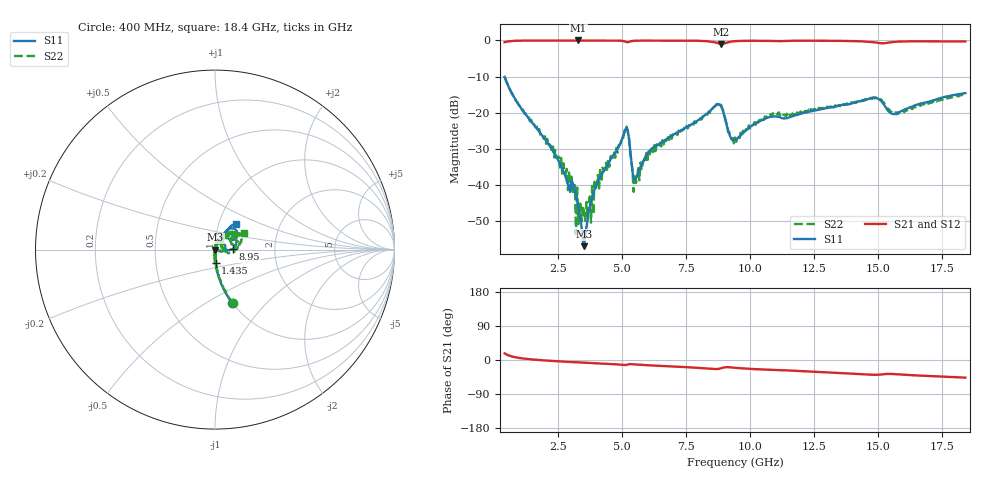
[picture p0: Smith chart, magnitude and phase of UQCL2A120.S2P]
! AVX Corporation
! Date:  10/27/06
! Part No:  UQCL2A120
! Description:  Ultra Low ESR Microwave capacitors
! Mounting Orientation:  Horizontal
# GHZ S DB R 50
! Freq  |S11|  S11 Ph  |S21|  S21 Ph  |S12|  S12 Ph  |S22|  S22 Ph
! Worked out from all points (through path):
!   401 points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, 400 MHz to 18.4 GHz, reference 50 ohm
!   highest |S21| = -0.02 dB at 3.28 GHz (marker M1); lowest = -1.0 dB at 8.86 GHz (marker M2)
!   group delay of S21, straight-line fit = 7.75 ps
!   lowest |S11| = -57.0 dB at 3.505 GHz (marker M3), VSWR 1.00, Z = 50.1 - j0.0112 ohm
!   |S11| at or under -10 dB: start of sweep to end of sweep
!   |S22| runs from -53.7 to -10.0 dB; largest |S21 - S12| = 0.0033
!   S11 on the Smith chart (normalised r, x): 400 MHz: 1.00, -0.66; 1.435 GHz: 1.00, -0.15; 8.95 GHz: 1.22, +0.01; 18.4 GHz: 1.21, +0.36
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0.4  -10.11 -72.1  -0.49 17.5  -0.48 17.4  -10.03 -71.0
1.435  -22.43 -87.4  -0.04 1.7  -0.03 1.7  -21.98 -87.6
2.695  -36.15 -91.3  -0.02 -4.2  -0.01 -4.2  -34.02 -94.8
2.875  -39.84 -98.1  -0.02 -4.9  -0.01 -4.9  -41.47 -87.0
3.1  -40.20 -86.7  -0.03 -5.7  -0.02 -5.7  -42.53 -126.5
3.28  -45.98 -81.4  -0.02 -6.3  -0.02 -6.3  -50.87 -14.1
3.415  -52.16 -62.8  -0.03 -6.8  -0.02 -6.8  -50.16 -179.6
3.505  -56.98 -4.5  -0.02 -7.1  -0.02 -7.1  -47.63 91.4
3.955  -40.70 67.0  -0.03 -8.5  -0.03 -8.6  -40.91 111.9
5.125  -24.55 35.0  -0.36 -13.3  -0.35 -13.4  -25.18 42.3
5.215  -25.08 1.3  -0.50 -11.7  -0.50 -11.8  -25.74 8.8
5.485  -38.65 23.5  -0.10 -11.9  -0.10 -11.9  -37.05 23.8
6.43  -28.71 66.9  -0.05 -15.4  -0.05 -15.4  -28.99 66.8
8.86  -18.32 13.6  -0.99 -21.7  -1.00 -21.8  -17.85 4.0
8.95  -20.01 2.3  -0.92 -19.9  -0.92 -20.0  -19.59 -9.2
9.22  -26.71 10.6  -0.36 -19.5  -0.37 -19.6  -27.00 5.3
9.4  -27.58 34.5  -0.22 -20.6  -0.23 -20.7  -26.88 23.9
10.795  -21.16 55.4  -0.16 -26.2  -0.16 -26.3  -20.39 52.8
12.415  -19.57 59.9  -0.10 -30.7  -0.10 -30.8  -19.52 53.5
14.845  -15.95 42.6  -0.55 -39.1  -0.55 -39.1  -16.05 29.0
15.43  -19.87 32.7  -0.58 -36.7  -0.59 -36.7  -19.12 13.2
18.4  -14.61 50.2  -0.29 -46.5  -0.30 -46.5  -14.74 29.7
